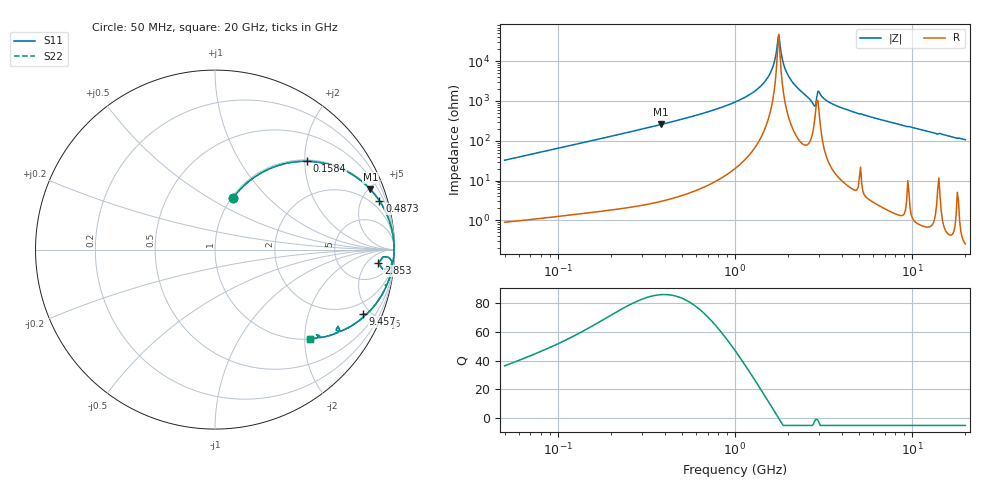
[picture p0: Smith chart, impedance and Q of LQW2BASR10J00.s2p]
!Murata Part Number: LQW2BASR10J00
!These Parameters are Measured in Series Mode Connection
!  o--[Z]--o
!Port1  Port2
!  o-------o
!Freq. Start=50[MHz] Stop=20[GHz], 401[Steps]
# Hz S RI R 50
!Freq.(Hz) S11(Real) S11(Imag) S21(Real) S21(Imag) S12(Real) S12(Imag) S22(Real) S22(Imag)
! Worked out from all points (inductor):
!   401 points, 50 MHz to 20 GHz, reference 50 ohm
!   read as one part in series: L = 103 nH near 51.52 MHz
!   highest Q = 85.6 at 383.4 MHz (marker M1), where L = 107 nH
!   self-resonance near 1.741 GHz
!   S11 on the Smith chart (normalised r, x): 50 MHz: 1.02, +0.65; 158.4 MHz: 1.03, +2.05; 487.3 MHz: 1.08, +6.74; 2.853 GHz: 12, -11; 9.457 GHz: 1.20, -4.49; 20 GHz: 1.01, -2.12
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5e7  0.1018 0.289  0.8982 -0.289  0.8982 -0.289  0.1018 0.289
1.364002e8  0.4388 0.488  0.5612 -0.488  0.5612 -0.488  0.4388 0.488
1.584406e8  0.5127 0.4921  0.4873 -0.4921  0.4873 -0.4921  0.5127 0.4921
3.721004e8  0.8583 0.3429  0.1417 -0.3429  0.1417 -0.3429  0.8583 0.3429
3.834161e8  0.866 0.3349  0.134 -0.3349  0.134 -0.3349  0.866 0.3349
4.872511e8  0.9164 0.2709  0.0836 -0.2709  0.0836 -0.2709  0.9164 0.2709
1e9  0.9865 0.1051  0.0135 -0.1051  0.0135 -0.1051  0.9865 0.1051
1.270815e9  0.9943 0.0594  0.00568 -0.0594  0.00568 -0.0594  0.9943 0.0594
1.476162e9  0.9969 0.0321  0.00313 -0.0321  0.00313 -0.0321  0.9969 0.0321
1.614971e9  0.9977 0.016  0.00235 -0.016  0.00235 -0.016  0.9977 0.016
1.714689e9  0.9979 0.00518  0.00213 -0.00518  0.00213 -0.00518  0.9979 0.00518
1.766834e9  0.9979 -0.000227  0.00212 0.000227  0.00212 0.000227  0.9979 -0.000227
1.820564e9  0.9978 -0.00566  0.00216 0.00566  0.00216 0.00566  0.9978 -0.00566
1.904239e9  0.9976 -0.0139  0.00236 0.0139  0.00236 0.0139  0.9976 -0.0139
2.021818e9  0.9971 -0.0251  0.00286 0.0251  0.00286 0.0251  0.9971 -0.0251
2.728004e9  0.9731 -0.1024  0.0269 0.1024  0.0269 0.1024  0.9731 -0.1024
2.853386e9  0.9108 -0.075  0.0892 0.075  0.0892 0.075  0.9108 -0.075
3.029571e9  0.9842 -0.0646  0.0158 0.0646  0.0158 0.0646  0.9842 -0.0646
3.850025e9  0.9789 -0.1357  0.0211 0.1357  0.0211 0.1357  0.9789 -0.1357
7.442007e9  0.8972 -0.3008  0.1028 0.3008  0.1028 0.3008  0.8972 -0.3008
9.457416e9  0.8243 -0.3589  0.1757 0.3589  0.1757 0.3589  0.8243 -0.3589
2e10  0.5286 -0.498  0.4714 0.498  0.4714 0.498  0.5286 -0.498
